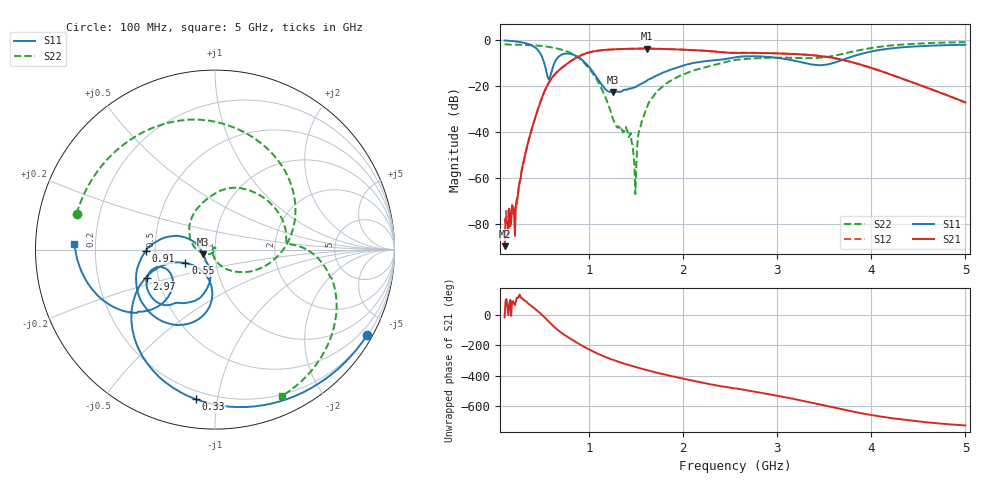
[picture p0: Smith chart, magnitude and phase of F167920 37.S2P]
!  2-Port S-parameters saved by WinCal
! VAR MeasName=S-Parameters (CALIBRATED_DATA) read from VNA (N5242A)
! VAR MeasDate=2016-11-22 9:57:14
! VAR NAME=F167920 37
! VAR FILENAME=F167920 37.S2P
! VAR DATE=2016-11-22 9:57:14
! VAR PHYS_PORTS=1,2
# Hz S DB R 50
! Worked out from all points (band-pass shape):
!   491 points, 100 MHz to 5 GHz, reference 50 ohm
!   highest |S21| = -3.78 dB at 1.61 GHz (marker M1); lowest = -89.8 dB at 100 MHz (marker M2)
!   |S21| within 3 dB of the highest: 910.9 MHz to 3.399 GHz (2.488 GHz wide, 115 % of centre)
!   lowest |S11| = -22.8 dB at 1.25 GHz (marker M3), VSWR 1.16, Z = 43.7 - j2.36 ohm
!   |S11| at or under -10 dB: 520.5 MHz to 630.4 MHz (109.9 MHz wide, 19.1 % of centre); 958 MHz to 2.117 GHz (1.159 GHz wide, 75.4 % of centre); 3.281 GHz to 3.601 GHz (319.9 MHz wide, 9.3 % of centre)
!   |S22| runs from -67.2 to -0.9 dB; largest |S21 - S12| = 0.002
!   S11 on the Smith chart (normalised r, x): 100 MHz: 0.22, -3.82; 330 MHz: 0.15, -0.87; 550 MHz: 0.71, -0.11; 910 MHz: 0.44, -0.01; 2.97 GHz: 0.43, -0.17; 5 GHz: 0.12, +0.02
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1e8  -0.25 -29.3  -89.83 -16.5  -77.96 109.2  -1.98 165.5
2.1e8  -0.63 -60.9  -85.38 63.4  -74.59 98.0  -2.06 149.3
3.3e8  -1.50 -97.1  -47.90 88.1  -48.24 87.6  -2.21 130.7
4.5e8  -4.26 -139.6  -30.75 26.7  -30.75 26.8  -2.47 110.1
5.5e8  -14.87 -155.8  -20.16 -32.4  -20.15 -32.4  -2.92 90.7
6.1e8  -12.21 -93.3  -16.19 -69.3  -16.18 -69.3  -3.35 78.3
7e8  -6.56 -116.5  -12.45 -115.1  -12.43 -115.0  -4.17 57.8
9.1e8  -8.26 -178.7  -6.79 163.7  -6.79 163.7  -8.63 -2.1
9.2e8  -8.53 178.7  -6.59 160.3  -6.58 160.2  -9.01 -5.4
1.11e9  -18.10 159.8  -4.59 100.5  -4.59 100.5  -19.52 -66.2
1.25e9  -22.83 -158.2  -4.15 66.1  -4.14 66.1  -34.21 -133.9
1.42e9  -21.22 -124.1  -3.91 31.6  -3.91 31.6  -42.34 83.6
1.49e9  -20.55 -113.5  -3.81 19.1  -3.81 19.1  -67.15 -0.7
1.54e9  -19.45 -107.2  -3.80 10.3  -3.79 10.3  -38.78 -123.8
1.61e9  -17.82 -100.6  -3.78 -1.6  -3.77 -1.6  -29.86 -136.7
1.74e9  -15.09 -99.1  -3.90 -21.9  -3.89 -21.9  -21.78 -170.1
2.11e9  -10.04 -113.2  -4.44 -72.7  -4.43 -72.7  -13.34 128.1
2.55e9  -7.60 -132.2  -5.66 -120.9  -5.64 -121.0  -8.79 71.4
2.97e9  -7.69 -157.0  -5.84 -166.5  -5.83 -166.7  -7.74 27.0
3.37e9  -10.73 -157.9  -6.66 144.0  -6.63 143.9  -7.92 5.5
4.19e9  -3.81 -149.9  -14.87 45.8  -14.86 45.4  -2.50 -25.3
5e9  -2.12 177.6  -27.26 -4.4  -27.26 -4.8  -0.94 -65.4
